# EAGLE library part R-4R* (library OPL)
Resistor Array
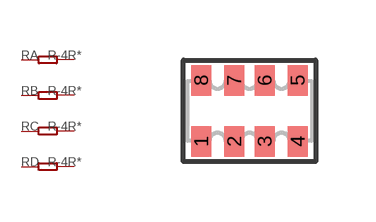
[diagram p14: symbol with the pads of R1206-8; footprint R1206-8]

Designator prefix R; gates A=R-1 B=R-1 C=R-1 D=R-1

## R-4R  [R1206-8]
1  A:1  pas
2  B:1  pas
3  C:1  pas
4  D:1  pas
5  D:2  pas
6  C:2  pas
7  B:2  pas
8  A:2  pas

## Footprint R1206-8 (pad centres in mm)
BOURNS Chip Resistor Array Source: RS Component / BUORNS
smd 0.508 x 0.762: 1 -1.206,-0.762; 2 -0.381,-0.762; 3 0.381,-0.762; 4 1.206,-0.762; 5 1.206,0.762; 6 0.381,0.762; 7 -0.381,0.762; 8 -1.206,0.762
